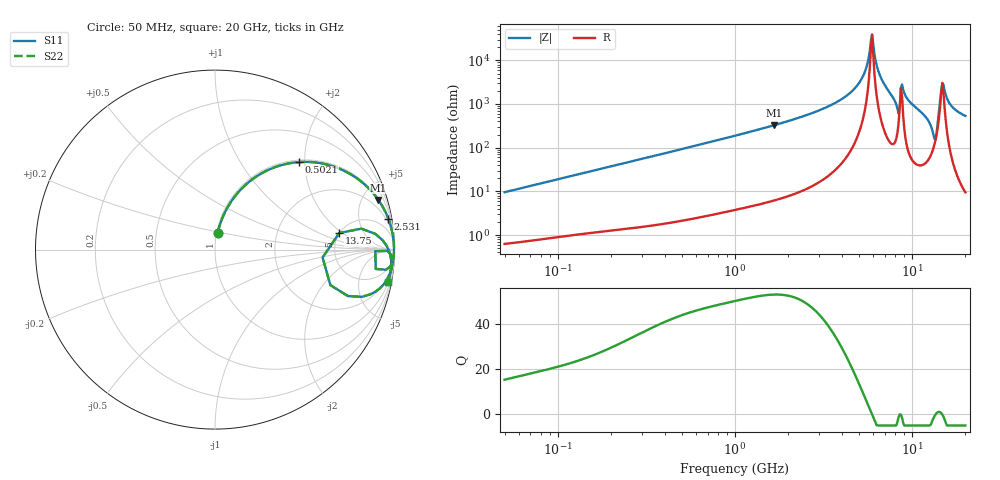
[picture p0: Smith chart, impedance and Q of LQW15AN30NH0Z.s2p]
!Murata Part Number: LQW15AN30NH0Z
!These Parameters are Measured in Series Mode Connection
!  o--[Z]--o
!Port1  Port2
!  o-------o
!Freq. Start=50[MHz] Stop=20[GHz], 401[Steps]
# Hz S RI R 50
!Freq.(Hz) S11(Real) S11(Imag) S21(Real) S21(Imag) S12(Real) S12(Imag) S22(Real) S22(Imag)
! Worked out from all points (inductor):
!   401 points, 50 MHz to 20 GHz, reference 50 ohm
!   read as one part in series: L = 30.3 nH near 51.52 MHz
!   highest Q = 52.9 at 1.664 GHz (marker M1), where L = 31.3 nH
!   self-resonance near 5.856 GHz
!   S11 on the Smith chart (normalised r, x): 50 MHz: 1.01, +0.19; 502.1 MHz: 1.04, +1.86; 2.531 GHz: 1, +11; 13.75 GHz: 4.96, +1.79; 20 GHz: 1, -11
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5e7  0.0151 0.0936  0.9849 -0.0936  0.9849 -0.0936  0.0151 0.0936
1.364002e8  0.0701 0.2356  0.9299 -0.2356  0.9299 -0.2356  0.0701 0.2356
3.721004e8  0.3271 0.4567  0.6729 -0.4567  0.6729 -0.4567  0.3271 0.4567
5.020686e8  0.4658 0.4875  0.5342 -0.4875  0.5342 -0.4875  0.4658 0.4875
1e9  0.7752 0.4076  0.2248 -0.4076  0.2248 -0.4076  0.7752 0.4076
1.664083e9  0.9105 0.2762  0.0895 -0.2762  0.0895 -0.2762  0.9105 0.2762
2.531158e9  0.9654 0.1728  0.0346 -0.1728  0.0346 -0.1728  0.9654 0.1728
2.728004e9  0.9716 0.1559  0.0284 -0.1559  0.0284 -0.1559  0.9716 0.1559
4.748272e9  0.9957 0.0433  0.00434 -0.0433  0.00434 -0.0433  0.9957 0.0433
5.352748e9  0.9971 0.0202  0.00285 -0.0202  0.00285 -0.0202  0.9971 0.0202
5.944466e9  0.9975 -0.000462  0.00251 0.000462  0.00251 0.000462  0.9975 -0.000462
6.503449e9  0.9969 -0.0192  0.00306 0.0192  0.00306 0.0192  0.9969 -0.0192
7.442007e9  0.9933 -0.0525  0.00668 0.0525  0.00668 0.0525  0.9933 -0.0525
8.264682e9  0.9531 -0.1119  0.0469 0.1119  0.0469 0.1119  0.9531 -0.1119
8.907419e9  0.9865 -0.044  0.0135 0.044  0.0135 0.044  0.9865 -0.044
1.276073e10  0.8657 -0.2493  0.1343 0.2493  0.1343 0.2493  0.8657 -0.2493
1.334722e10  0.6428 -0.1977  0.3572 0.1977  0.3572 0.1977  0.6428 -0.1977
1.375312e10  0.6924 0.0925  0.3076 -0.0925  0.3076 -0.0925  0.6924 0.0925
1.460232e10  0.9569 0.0198  0.0431 -0.0198  0.0431 -0.0198  0.9569 0.0198
1.504638e10  0.9756 -0.0265  0.0244 0.0265  0.0244 0.0265  0.9756 -0.0265
1.670968e10  0.9806 -0.1083  0.0194 0.1083  0.0194 0.1083  0.9806 -0.1083
2e10  0.9633 -0.1794  0.0367 0.1794  0.0367 0.1794  0.9633 -0.1794
